(* Logix 5000 AddOnInstructionDefinition export T2STA; software revision 32.02 *)

TYPE Exlar_Control :   // Tritex II Control
STRUCT
   EnableOutputs : INT;   // EnableOutputs
   InputEventsMode : INT;   // 4316
   InputEventsModeLevel : INT;   // 4318
   InputEventsMotion : INT;   // 4317
   HostCommandControlMode : INT;   // 4303
   HostPosition_low : INT;   // 4304
   HostPosition_high : INT;
   HostVelocity_low : INT;   // 4306
   HostVelocity_high : INT;
   HostAcceleration_low : INT;   // 4308
   HostAcceleration_high : INT;
   HostCurrent : INT;   // 4310
   InputEventsMoveEdge : INT;   // 4319
   JogSlowVelocity_low : INT;   // 6022
   JogSlowVelocity_high : INT;
   JogAcceleration_low : INT;   // 6026
   JogAcceleration_high : INT;
   MoveOption : INT;   // 6100
   MoveCurrentLimit : INT;   // 6101
   MoveAcceleration_low : INT;   // 6102
   MoveAcceleration_high : INT;
   MoveDeceleration_low : INT;   // 6500
   MoveDeceleration_high : INT;
   MovePrimaryOption : INT;   // 6106
   spare : INT;   // spare
   MovePrimaryPosition_low : INT;   // 6108
   MovePrimaryPosition_high : INT;
   MovePrimaryVelocity_low : INT;   // 6110
   MovePrimaryVelocity_high : INT;
   MoveSecondaryOption : INT;   // 6112
   spare2 : INT;   // spare
   MoveSecondaryPosition_low : INT;   // 6114
   MoveSecondaryPosition_high : INT;
   MoveSecondaryVelocity_low : INT;   // 6116
   MoveSecondaryVelocity_high : INT;
END_STRUCT
END_TYPE

TYPE Exlar_Drive :   // Tritex II Data
STRUCT
   Control : Exlar_Control;   // Control bits to send to the drive
   Status : Exlar_Status;   // Status bits received from the drive
END_STRUCT
END_TYPE

TYPE Exlar_Status :   // Tritex II Status
STRUCT
   EIP_Comm : INT;   // EIP module communication
   OutputEventsStatus : INT;   // 104
   OutputEventsMoveInPosition : INT;   // 108
   OutputEventsMotion : INT;   // 105
   OutputsEventsMotionActive : INT;   // 107
   PositionFeedback_low : INT;   // 378
   PositionFeedback_high : INT;
   SoftFaults : INT;   // 7
   HardFaults : INT;   // 6
   VelocityDisplay_low : INT;   // 356
   VelocityDisplay_high : INT;
   CurrentDisplay : INT;   // 567
   CurrentContinuous : INT;   // 565
   CurrentLimit : INT;   // 5108
   VoltageHallBattery : INT;   // 8
   VoltageBus : INT;   // 571
   TemperatureBoard : INT;   // 11
   TemperatureActuator : INT;   // 15
END_STRUCT
END_TYPE

ADD_ON_INSTRUCTION T2STA   (* revision 1.0, vendor Exlar Corporation *)
// Help:
// Use the Tritex 2 Status (T2STA) instruction to retrieve drive status. The instruction parameters provide a summary view of the module, motion and position information for the drive.
// Configured for Exlar EIP AOI. 07/01/2014
// ----------------------------------------------------------------------------------------------------------------------------
// Parameters Bit Definition
// ----------------------------------------------------------------------------------------------------------------------------
// Module:   (Output) Module Status
// ------------------------------------------------------------------
//      Module.0:     Enable
//      Module.1:     Homed
//      Module.2:     Ready
//      Module.3:     Fault Active
//      Module.4:     Warning Active
//      Module.5:     Fault or Warning Active
// Motion:   (Output) Motion Status
// ------------------------------------------------------------------
//      Motion.0:     Stopped Active
//      Motion.1:     Pasued Active
//      Motion.2:     Jogged Active
//      Motion.3:     Jog Positive Active
//      Motion.4:     Jog Negative Active
//      Motion.5:     Initiate Home Move Active
//      Motion.6:     Emergency Move Active
//      Motion.7:     Move Active
//      Motion.8:     In Position Active
// Warnings:     (Output) List of active drive Warnings
// ------------------------------------------------------------------
//      Warnings.0:  IPK – Peak Current
//      Warnings.1:  C – Continuous Current
//      Warnings.2:  POS – Position Tracking
//      Warnings.3:  MV – Move Termination
//      Warnings.4:  VLOW – Low DC Bus Voltage
//      Warnings.5:  VHIGH – High DC Bus Voltage
//      Warnings.6:  FE – Positional Following Error
//      Warnings.7:  BT – Board Temperature
//      Warnings.8:  AT – Actuator Temperature
//      Warnings.9:  LOS – Loss of Signal
//      Warnings.10:  COM –Communications
//      Warnings.11:  IH – Hardware Over current
//      Warnings.12:  HB – Absolute Hall Board Battery
//      Warnings 13:  UP – User Parameters
//      Warnings.14:  FP – Factory Parameters
//      Warnings.15:  RS – Restart
// Faults:     (Output)  List of active drive Faults
// ------------------------------------------------------------------
//      Faults.0:  IPK – Peak Current
//      Faults.1:  C – Continuous Current
//      Faults.2:  POS – Position Tracking
//      Faults.3:  MV – Move Termination
//      Faults.4:  VLOW – Low DC Bus Voltage
//      Faults.5:  VHIGH – High DC Bus Voltage
//      Faults.6:  FE – Positional Following Error
//      Faults.7:  BT – Board Temperature
//      Faults.8:  AT – Actuator Temperature
//      Faults.9:  LOS – Loss of Signal
//      Faults.10:  COM –Communications
//      Faults.11:  IH – Hardware Over current
//      Faults.12:  HB – Absolute Hall Board Battery
//      Faults 13:  UP – User Parameters
//      Faults.14:  FP – Factory Parameters
//      Faults.15:  RS – Restart
VAR_IN_OUT
   Drive : Exlar_Drive; {required}   // Drive
   Units : REAL[5]; {required}   // User Units Configuration
END_VAR
VAR_OUTPUT
   DF : BOOL; {access Read Only, visible}   // A Drive Fault is active
   ER : BOOL; {access Read Only, visible}   // A Instruction error is Active
   Ready : BOOL; {access Read Only, visible}   // Enabled + Homed
   Module : INT; {access Read Only, visible}   // Drive Status
        .0   // Enable
        .1   // Homed
        .2   // Ready
        .3   // Fault
        .4   // Warning
        .5   // Fault or Warning
        .7   // Alternate Operating Mode
        .10   // Define Home Position 1
        .11   // Define Home Position 2
        .12   // Move Teach Enable
        .13   // Teach Selected Move Position
        .14   // Brake Override
        .15   // Fault Reset
   Motion : INT; {access Read Only, visible}   // Motion Status
        .0   // Stopped Active
        .1   // Pasued Active
        .2   // Jogged Active
        .3   // Jog Positive Actived
        .4   // Jog Negative Active
        .5   // Initiate Home Move Active
        .6   // EMOVE
        .7   // Move active
        .8   // In Position active
   Position : REAL; {access Read Only, visible}   // Module Position
   Velocity : REAL; {access Read Only, visible}   // Module Velocity
   ContinuousCurrent : REAL; {access Read Only, visible}   // Continous Current
   ActualCurrent : REAL; {access Read Only, visible}   // Actual Current
   Battery : INT; {access Read Only, visible}   // Battery Voltage if available
   BusVoltage : INT; {access Read Only, visible}   // Bus Voltage
   BoardTemp : INT; {access Read Only, visible}   // Board Temperature
   ActuatorTemp : INT; {access Read Only, visible}   // Actuator Temperature
   Warnings : INT; {access Read Only, visible}   // Warnings
        .0   // IPK- Peak Current
        .1   // C - Continuous Current
        .2   // POS - Position Tracking
        .3   // MV - Move Termination
        .4   // VLOW - Low DC Bus Voltage
        .5   // VHIGH - High DC Bus Voltage
        .6   // FE - Positional Following Error
        .7   // BT - Board Temperature
        .8   // AT - Actuator Temperature
        .9   // LOS - Loss of Signal
        .10   // COM - Communications
        .11   // IH - Hardware Over current
        .12   // AB- Absolute Hall Board Battery
        .13   // UP - User Parameters
        .14   // FP - Factory Parameters
        .15   // RS - Restart
   Faults : INT; {access Read Only, visible}   // Faults
        .0   // IPK- Peak Current
        .1   // C - Continuous Current
        .2   // POS - Position Tracking
        .3   // MV - Move Termination
        .4   // VLOW - Low DC Bus Voltage
        .5   // VHIGH - High DC Bus Voltage
        .6   // FE - Positional Following Error
        .7   // BT - Board Temperature
        .8   // AT - Actuator Temperature
        .9   // LOS - Loss of Signal
        .10   // COM - Communications
        .11   // IH - Hardware Over current
        .12   // HB - Absolute Hall Board Battery
        .13   // UP - User Parameters
        .14   // FP - Factory Parameters
        .15   // RS - Restart
END_VAR
VAR
   tempDINT : DINT; {access None}   // Temporary Register used in calculating units
END_VAR

ROUTINE Logic   (* structured text *)
   (***********************************************)
   (*   Exlar Tritex 2 Status                     *)
   (*                                             *)
   (***********************************************)
   
   (*********** OUTPUTS  ***********)
   
   (* Drive Faults Active *)
   	(* 104.03 Fault *)
   	If Drive.Status.OutputEventsStatus.3 then
    		DF := 1;
   	Else
   		DF := 0;
   	End_If;
   
   (* Ready Active *)
   	(* 104.02 Ready *)
   	if Drive.Status.OutputEventsStatus.2 then
   		Ready := 1;
   	else
   		Ready := 0;
   	End_if;
   
   (* Drive Warnings Active *)
   (* ID:7, Status.Mode.SoftFaults : ModuleInputs[7]*)
   	Warnings := Drive.Status.SoftFaults;
   
   (* Drive Faults Active *)
   (* ID:6, Status.Mode.HardFaults : ModuleInputs[8]*)
   	Faults := Drive.Status.HardFaults;
   
   (* Module  *)
   	(* 104.00 Enable *)
   	(* 104.01 Homed *)
   	(* 104.02 Ready *)
   	(* 104.03 Fault *)
   	(* 104.04 Warning *)
   	(* 104.05 Fault or Warning *)
   	Module := Drive.Status.OutputEventsStatus AND 16#3F;
   
   (* Motion *)
   	(* 105.00 Stopped Active *)
   	If Drive.Status.OutputEventsMotion.0 Then
   		Motion.0 := 1;
   	else
   		Motion.0 := 0;
   	end_if;
   
   	(* 105.01 Pause *)
   	If Drive.Status.OutputEventsMotion.1 Then
   		Motion.1 := 1;
   	else
   		Motion.1 := 0;
   	end_if;
   
   	(* 105.02 Jogging *)
   	If Drive.Status.OutputEventsMotion.2 Then
   		Motion.2 := 1;
   	else
   		Motion.2 := 0;
   	end_if;
   
   	(* 105.03 Jogging Plus *)
   	If Drive.Status.OutputEventsMotion.3 Then
   		Motion.3 := 1;
   	else
   		Motion.3 := 0;
   	end_if;
   
   	(* 105.04 Jogging Minus *)
   	If Drive.Status.OutputEventsMotion.4 Then
   		Motion.4 := 1;
   	else
   		Motion.4 := 0;
   	end_if;
   
   	(* 105.05 Homing Active *)
   	If Drive.Status.OutputEventsMotion.5 Then
   		Motion.5 := 1;
   	else
   		Motion.5 := 0;
   	end_if;
   
   	(* 105.08 Dedicated Move Active *)
   	If Drive.Status.OutputEventsMotion.8 Then
   		Motion.6 := 1;
   	else
   		Motion.6 := 0;
   	end_if;
   
   	(* 105.09 Move Active *)
   	If Drive.Status.OutputEventsMotion.9 Then
   		Motion.7 := 1;
   	else
   		Motion.7 := 0;
   	end_if;
   
   	(* 105.12 Input Position *)
   	If Drive.Status.OutputEventsMotion.12 Then
   		Motion.8 := 1;
   	else
   		Motion.8 := 0;
   	end_if;
   
   (* Units  *)
   	IF Units[0] = 0 THEN
   		ER := 1;
   	else
   		ER := 0;
   
   		(* Velocity *)
   		(*  ID:356, Status.Velocity.Display:    ModuleInputs[10],ModuleInputs[9] *)
   		cps(Drive.Status.VelocityDisplay_low,tempDINT,2);
   		Velocity    :=  tempDINT * Units[2];
   
   		(* Position *)
   		(*	ID:378, Status.Position.Feedback:   ModuleInputs[6],ModuleInputs[5]  *)
   		cps(Drive.Status.PositionFeedback_low,tempDINT,2);
   		Position	:=	tempDINT * Units[1];
   
   		(* Current scale ? *)
   		(*       0: AMPs   *)
   		(*       1: %      *)
   		if Units[4] = 0	then
   			(* ID:567, Status.Current.Display:  ModuleInputs[11]  *)
   			ActualCurrent := Drive.Status.CurrentDisplay * 0.0078125;
   
   			(* ID:565, Status.Current.Continuous:  ModuleInputs[12]*)
   			ContinuousCurrent := Drive.Status.CurrentContinuous * 0.0078125;
   		else
   			(* Use for %,ID:5108, Config.CurrentLimit:   ModuleInputs[13],  *)
   			ActualCurrent  :=  (Drive.Status.CurrentDisplay / Drive.Status.CurrentLimit) * 100;
   			ContinuousCurrent :=  (Drive.Status.CurrentContinuous / Drive.Status.CurrentLimit) * 100;
   		end_if;
   	end_if;
   
   (*	ID:15,  Status.Temperature.Actuator:ModuleInputs[17] *)
    	ActuatorTemp 	:=	Drive.Status.TemperatureActuator * 0.125;
   (*	ID:11,  Status.Temperature.Board: 	ModuleInputs[16] *)
   	BoardTemp		:=	Drive.Status.TemperatureBoard * 0.03125;
   (*	ID:571, Status.Voltage.Vbus:    	ModuleInputs[15] *)
   	BusVoltage		:=	Drive.Status.VoltageBus *  0.03125;
   (*	ID:08,  Status.Voltage.HallBattery: ModuleInputs[14] *)
   
   
END_ROUTINE
END_ADD_ON_INSTRUCTION
